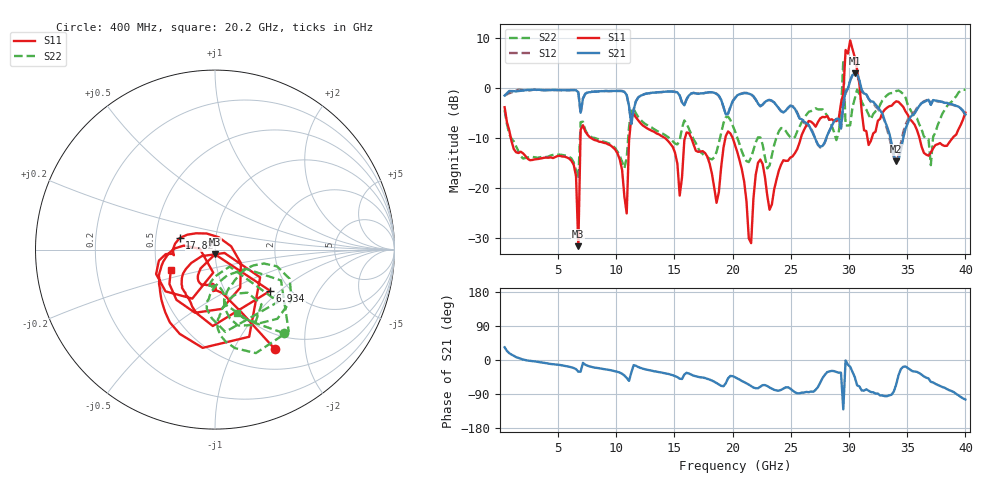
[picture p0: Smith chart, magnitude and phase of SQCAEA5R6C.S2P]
! Network Analyzer HP8722ES.07.66: Jul 25, 2000 Serial No. US39175408
! 26 Oct 2004  15:11:17
! Frequency  S11  S21  S12  S22
# HZ  S  DB R  50
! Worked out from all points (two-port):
!   201 points, 400 MHz to 40 GHz, reference 50 ohm
!   highest |S21| = 2.90 dB at 30.5 GHz (marker M1); lowest = -14.6 dB at 34.06 GHz (marker M2)
!   |S21| within 3 dB of the highest: 29.9 GHz to 31.06 GHz (1.158 GHz wide, 3.8 % of centre)
!   lowest |S11| = -31.5 dB at 6.736 GHz (marker M3), VSWR 1.05, Z = 49.9 - j2.65 ohm
!   |S11| at or under -10 dB: 939.2 MHz to 6.92 GHz (5.98 GHz wide, 152 % of centre); 7.849 GHz to 11.12 GHz (3.267 GHz wide, 34.5 % of centre); 20.01 GHz to 25.86 GHz (5.848 GHz wide, 25.5 % of centre)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
!   |S22| runs from -18.1 to 5.5 dB; largest |S21 - S12| = 0.14
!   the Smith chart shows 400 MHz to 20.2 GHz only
!   S11 on the Smith chart (normalised r, x): 400 MHz: 0.78, -1.47; 6.934 GHz: 1.60, -0.86; 17.82 GHz: 0.67, +0.09; 20.2 GHz: 0.59, -0.15
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4e8  -3.82 -59.0  -1.49 33.5  -1.52 37.6  -4.42 -50.6
6.736e9  -31.54 -89.8  -0.83 -30.9  -0.86 -31.3  -18.07 -49.1
6.934e9  -8.32 -36.7  -4.93 -30.6  -5.18 -29.8  -6.80 -39.5
7.132e9  -7.41 -91.7  -2.12 -7.6  -2.06 -8.3  -6.71 -82.9
1.0894e10  -25.01 -19.5  -1.37 -47.5  -1.40 -48.0  -13.90 -31.9
1.129e10  -5.65 -68.6  -7.17 -33.0  -7.18 -31.7  -4.25 -47.9
1.3666e10  -9.24 -155.0  -0.83 -32.1  -0.82 -31.9  -8.73 -85.9
1.7824e10  -13.68 161.9  -0.89 -49.6  -0.91 -49.4  -13.82 -57.4
2.02e10  -11.34 -155.2  -2.04 -45.3  -1.92 -45.1  -8.59 -70.8
2.1586e10  -30.94 12.6  -1.30 -68.9  -1.24 -68.5  -13.85 -30.6
2.6932e10  -7.11 -64.6  -9.23 -83.9  -9.04 -83.4  -4.32 -3.6
2.9308e10  -3.03 -15.9  -8.07 -33.5  -8.04 -32.5  -5.09 13.0
2.9506e10  -1.10 7.2  -3.15 -130.3  -3.95 -119.4  5.52 48.8
2.9704e10  7.59 16.4  -0.68 -1.0  -1.10 6.3  -7.47 -53.6
2.9902e10  6.87 -61.6  -0.11 -12.3  -0.08 -12.0  -7.46 14.5
3.01e10  9.49 -76.7  1.48 -17.8  1.51 -17.9  -7.42 23.1
3.0496e10  6.14 -104.0  2.90 -45.1  2.82 -45.2  -2.10 0.8
3.0694e10  3.67 45.7  2.84 -66.8  2.69 -65.2  -0.29 163.8
3.1486e10  -8.60 -113.1  -1.24 -77.4  -1.26 -78.1  -4.32 -30.9
3.3466e10  -3.62 -67.5  -9.08 -93.3  -9.84 -91.0  -1.09 -15.5
3.406e10  -2.65 -82.3  -14.65 -63.8  -14.55 -54.3  -0.58 -27.5
4e10  -4.90 -59.7  -5.28 -104.3  -5.35 -103.3  -0.35 1.4
